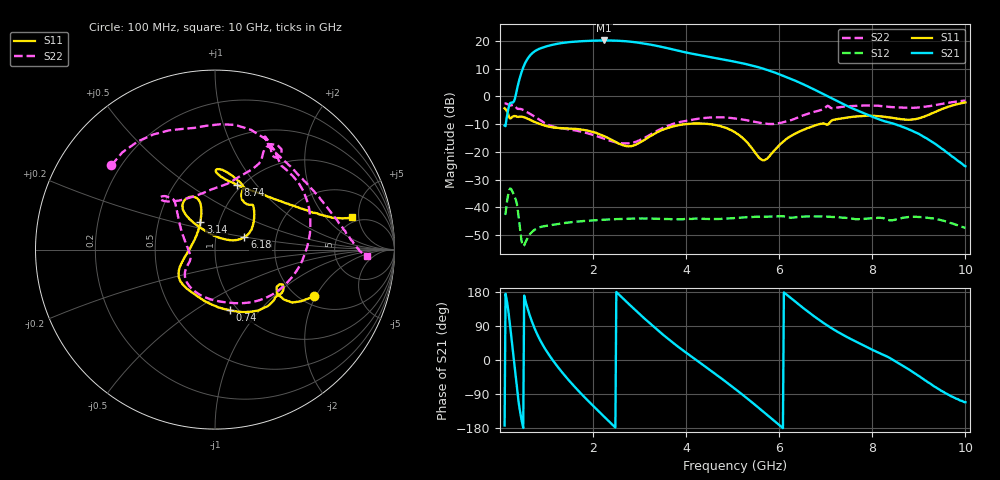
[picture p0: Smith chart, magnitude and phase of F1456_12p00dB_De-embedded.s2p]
! Integrated Device Technology
! Corporate Headquarters
! 6024 Silver Creek Valley Road
! San Jose, CA 95138  USA
! Phone:  1-408-284-8200
! Toll Free:  1-800-223-1366
! Webpage:  http://www.idt.com/
! Timing and RF Division
! 515 Groton Road, Suite 102
! Westford, MA 01886-6024
! Device:  F1456
! Description: 6-bit 0.5 dB Transmit Variable Gain Amplifier
! Frequency:  2100.0 -  2950.00 MHz
! Package:  6x6 mm Thin QFN Plastic Package: 28 pin
! State:  24
! Atten State:  12.0 dB
! Voltage:  +5.00 Volts
! Current:  217.029 mA
! Data:  The device was measured on a the F1455 evaluation board which has
!  individual transmission lines to the RF pins.  Data was collected
!  using a calibrated network analyzer.  The evaluation board was
!  de-embedded using a TRL calibration technique.
!  The reference plane is the edge of the package pin.
!  Pin  1 = CSb
!  Pin  2 = DATA
!  Pin  3 = CLK
!  Pin  4 = RSET
!  Pin  5 = GND
!  Pin  6 = RFIN  = Port 1
!  Pin  7 = GND
!  Pin  8 = NC
!  Pin  9 = NC
!  Pin 10 = NC
!  Pin 11 = NC
!  Pin 12 = NC
!  Pin 13 = NC
!  Pin 14 = /STBY
!  Pin 15 = GND
!  Pin 16 = RFOUT  = Port 2
!  Pin 17 = GND
!  Pin 18 = NC
!  Pin 19 = NC
!  Pin 20 = NC
!  Pin 21 = GND
!  Pin 22 = NC
!  Pin 23 = GND
!  Pin 24 = NC
!  Pin 25 = NC
!  Pin 26 = NC
!  Pin 27 = GND
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# GHz S dB R 50
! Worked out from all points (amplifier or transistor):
!   496 points, 100 MHz to 10 GHz, reference 50 ohm
!   highest |S21| = 20.2 dB at 2.24 GHz (marker M1)
!   |S21| within 3 dB of that: 847.5 MHz to 3.653 GHz (2.805 GHz wide, 125 % of centre)
!   unconditionally stable (mu >= 1): start of sweep to end of sweep
!   at 1.74 GHz: K = 8.04, MAG = 20.4 dB, |S12| = -45.0 dB
!   at 5.06 GHz: K = 14.78, MAG = 13.5 dB, |S12| = -43.9 dB
!   at 10 GHz: K = 238.01, MAG = -15.6 dB, |S12| = -47.5 dB
!   S11 on the Smith chart (normalised r, x): 100 MHz: 2.34, -1.95; 740 MHz: 0.92, -0.71; 3.14 GHz: 0.81, +0.25; 6.18 GHz: 1.37, +0.19; 8.74 GHz: 0.95, +0.80; 10 GHz: 4.31, +4.03
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0.1  -4.26 -25.2  -10.50 -172.9  -42.28 47.0  -2.57 140.9
0.32  -7.06 -32.4  -0.87 -21.0  -36.40 -142.7  -3.37 65.8
0.44  -7.28 -42.5  7.48 -142.1  -49.03 139.2  -4.49 38.7
0.58  -7.91 -59.1  13.25 141.7  -51.50 171.4  -5.62 5.4
0.74  -9.15 -76.1  16.23 84.8  -48.15 136.9  -7.19 -26.7
0.96  -10.49 -97.3  17.89 31.5  -46.78 94.7  -9.58 -64.1
1.18  -11.26 -114.6  18.84 -8.2  -46.25 68.5  -11.00 -91.5
1.48  -11.53 -131.5  19.61 -53.6  -45.46 42.4  -11.87 -119.4
1.76  -11.94 -143.1  19.96 -90.9  -45.00 23.4  -12.75 -135.8
2.24  -14.31 -160.4  20.22 -149.7  -44.47 -4.1  -15.24 -151.0
2.64  -17.57 169.8  20.01 162.9  -44.18 -24.9  -16.93 -164.3
3.14  -15.26 118.3  19.00 105.5  -44.06 -50.2  -14.61 159.3
3.4  -12.76 109.2  18.16 77.5  -44.14 -62.5  -12.23 143.5
3.74  -10.71 108.3  16.88 43.4  -44.34 -77.0  -9.80 132.2
4.1  -9.80 114.5  15.52 10.4  -44.19 -92.1  -8.50 130.5
5.06  -13.02 129.9  12.51 -76.9  -43.86 -133.8  -7.92 137.0
5.64  -22.97 77.0  10.12 -134.6  -43.38 -165.4  -9.68 121.1
6.18  -15.03 22.8  6.79 170.4  -43.57 161.3  -8.87 83.0
6.7  -10.88 40.3  2.94 119.8  -43.28 134.2  -5.80 64.1
8.36  -7.53 87.6  -9.37 6.4  -44.65 63.6  -3.76 62.5
8.74  -8.37 71.0  -11.57 -21.4  -43.57 54.3  -4.08 49.2
10  -2.13 13.4  -25.19 -111.3  -47.46 -26.1  -1.46 -2.5
